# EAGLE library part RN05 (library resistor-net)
RESISTOR NETWORK
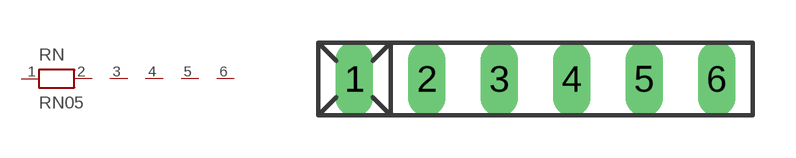
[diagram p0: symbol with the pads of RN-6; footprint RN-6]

Designator prefix RN

## RN05 (OC_FARNELL: unknown; OC_NEWARK: unknown)  [RN-6]
1  1  pas
2  2  pas
3  3  pas
4  4  pas
5  5  pas
6  6  pas

## Footprint RN-6 (pad centres in mm)
RESISTOR NETWORK
drill 0.813 long: 1 -6.35,0; 2 -3.81,0; 3 -1.27,0; 4 1.27,0; 5 3.81,0; 6 6.35,0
